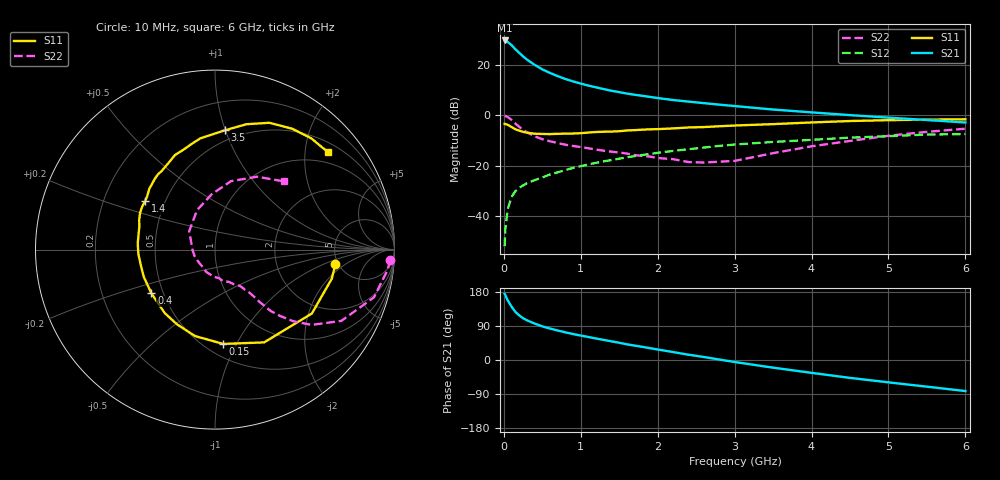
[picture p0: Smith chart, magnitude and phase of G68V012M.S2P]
! SIEMENS Small Signal Semiconductors
! BFG193
! Si NPN RF Bipolar Junction Transistor in SOT223
! VCE = 8 V  IC = 12 mA
! Common Emitter S-Parameters:  August  1996
# GHz  S  MA  R  50
!  f  S11  S21  S12  S22
! GHz  MAG  ANG  MAG  ANG  MAG  ANG  MAG  ANG
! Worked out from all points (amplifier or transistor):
!   36 points, 10 MHz to 6 GHz, reference 50 ohm
!   highest |S21| = 29.7 dB at 10 MHz (marker M1)
!   |S21| within 3 dB of that: start of sweep to 135.2 MHz
!   unconditionally stable (mu >= 1): 860.2 MHz to 2.485 GHz
!   at 250 MHz: K = 0.58, MSG = 25.7 dB, |S12| = -27.9 dB
!   at 1.4 GHz: K = 1.06, MAG = 12.3 dB, |S12| = -17.8 dB
!   at 6 GHz: K = 0.86, MSG = 2.3 dB, |S12| = -7.5 dB
!   S11 on the Smith chart (normalised r, x): 10 MHz: 4.72, -1.44; 150 MHz: 0.61, -0.89; 400 MHz: 0.43, -0.26; 1.4 GHz: 0.39, +0.27; 3.5 GHz: 0.42, +1.00; 6 GHz: 0.72, +2.52
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0.01  0.6763 -7.0  30.7 174.7  0.0025 96.7  0.9791 -3.4
0.02  0.6703 -14.1  30.37 171.1  0.0056 87.3  0.9671 -6.9
0.05  0.6466 -33.4  28.74 157.3  0.0135 74.6  0.9248 -16.7
0.1  0.5849 -62.1  24.79 141.0  0.0238 65.7  0.8086 -29.4
0.15  0.5276 -85.0  20.56 126.8  0.031 57.9  0.6831 -37.9
0.2  0.4944 -103.0  17.42 117.8  0.0362 55.0  0.591 -42.5
0.25  0.4671 -116.9  14.81 110.3  0.0403 53.0  0.5121 -45.8
0.3  0.4513 -128.3  12.82 104.7  0.0446 53.0  0.4607 -47.8
0.4  0.43 -145.5  10.06 96.2  0.0513 53.3  0.3823 -49.6
0.5  0.4249 -158.9  8.177 88.7  0.0581 53.3  0.3343 -50.5
0.6  0.4223 -168.5  6.937 83.0  0.0665 53.7  0.3044 -51.5
0.7  0.4277 -176.7  6.003 77.8  0.0734 54.1  0.2806 -53.2
0.9  0.4339 169.4  4.71 68.5  0.0898 53.0  0.2451 -55.6
1.1  0.4539 158.5  3.89 60.6  0.1055 51.8  0.2207 -61.3
1.4  0.4741 145.0  3.064 49.2  0.129 48.1  0.1889 -70.2
1.7  0.506 134.1  2.556 38.0  0.1541 44.0  0.1618 -81.4
2.2  0.5481 118.1  2.008 20.9  0.1957 34.6  0.134 -111.1
2.8  0.6048 102.0  1.627 1.3  0.246 22.7  0.1193 -160.5
3.5  0.6667 85.3  1.301 -20.2  0.295 6.6  0.1767 144.6
4.5  0.7687 66.8  1.007 -47.2  0.3598 -13.1  0.3089 93.4
5.5  0.8196 49.2  0.805 -70.4  0.4143 -37.1  0.4689 60.0
6  0.8317 40.6  0.719 -81.9  0.4227 -51.1  0.5402 44.7
